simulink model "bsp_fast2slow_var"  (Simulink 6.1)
settings: Solver=VariableStepDiscrete  StartTime=0.0  StopTime=20.0  RelTol=1e-3

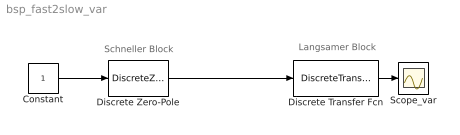
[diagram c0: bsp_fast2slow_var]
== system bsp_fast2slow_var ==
  note: Langsamer Block
  note: Schneller Block
  Constant : Constant
  Discrete Transfer Fcn : DiscreteTransferFcn  Denominator=[1 0.5 1]  SampleTime=2
  Discrete Zero-Pole : DiscreteZeroPole  Poles=[0 0 0.1]  Gain=2
  Scope_var : Scope
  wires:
  Discrete Transfer Fcn/1 -> Scope_var/1
  Constant/1 -> Discrete Zero-Pole/1
  Discrete Zero-Pole/1 -> Discrete Transfer Fcn/1
